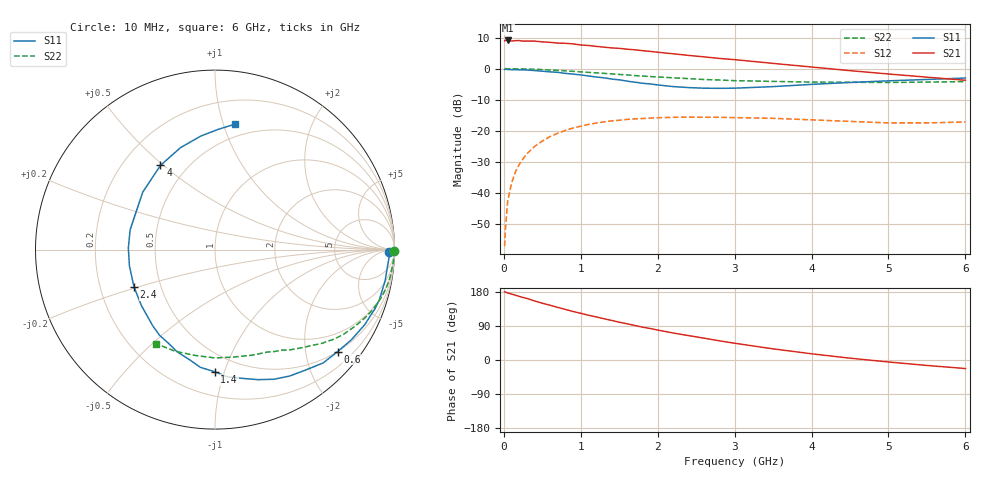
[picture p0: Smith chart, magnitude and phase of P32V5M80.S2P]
! SIEMENS Small Signal Semiconductors
! BFP181
! Si NPN RF Bipolar Junction Transistor in SOT143
! VCE = 2.5 V  IC = 0.8 mA
! Common Emitter S-Parameters:  March  1996
# GHz  S  MA  R  50
!  f  S11  S21  S12  S22
! GHz  MAG  ANG  MAG  ANG  MAG  ANG  MAG  ANG
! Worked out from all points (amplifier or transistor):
!   36 points, 10 MHz to 6 GHz, reference 50 ohm
!   highest |S21| = 9.1 dB at 50 MHz (marker M1)
!   |S21| within 3 dB of that: start of sweep to 1.697 GHz
!   unconditionally stable (mu >= 1): 3.36 GHz to end of sweep
!   at 250 MHz: K = 0.08, MSG = 18.9 dB, |S12| = -29.0 dB
!   at 1.4 GHz: K = 0.47, MSG = 11.7 dB, |S12| = -16.8 dB
!   at 6 GHz: K = 1.33, MAG = 3.3 dB, |S12| = -17.1 dB
!   S11 on the Smith chart (normalised r, x): 10 MHz: 54, -24; 600 MHz: 0.50, -2.68; 1.4 GHz: 0.37, -0.93; 2.4 GHz: 0.35, -0.19; 4 GHz: 0.36, +0.49; 6 GHz: 0.39, +1.09
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0.01  0.9696 -0.8  2.803 179.8  0.0014 87.9  0.999 -0.3
0.02  0.9785 -1.3  2.839 179.4  0.0026 91.6  0.9995 -0.7
0.05  0.97 -2.9  2.841 177.0  0.0074 90.7  0.9974 -1.6
0.1  0.9644 -6.8  2.782 174.1  0.0144 85.0  0.9969 -3.2
0.15  0.964 -10.2  2.816 171.0  0.0218 82.7  0.9943 -4.7
0.2  0.959 -13.4  2.827 167.9  0.0288 81.0  0.9914 -6.4
0.4  0.933 -26.7  2.776 155.8  0.0562 72.2  0.9776 -12.6
0.6  0.8887 -39.8  2.651 144.5  0.0809 63.2  0.9526 -18.4
0.8  0.84 -53.0  2.559 133.4  0.1018 54.8  0.9227 -23.8
0.9  0.8174 -59.6  2.499 128.1  0.1111 51.0  0.9044 -26.4
1.1  0.7631 -71.7  2.359 118.1  0.1268 43.9  0.8713 -31.2
1.4  0.6807 -90.1  2.156 104.5  0.1446 34.3  0.8243 -37.6
1.5  0.661 -97.1  2.123 99.8  0.1481 31.7  0.8064 -39.3
1.8  0.5828 -116.4  1.949 86.8  0.1579 24.2  0.7613 -44.4
2.2  0.515 -142.8  1.735 71.3  0.165 15.4  0.7127 -50.9
2.4  0.4967 -155.4  1.634 64.4  0.1664 11.4  0.6923 -54.0
3  0.4855 166.8  1.396 44.2  0.1633 2.3  0.6415 -62.8
3.5  0.5144 141.5  1.216 29.4  0.159 -2.8  0.6238 -70.5
4  0.5591 122.9  1.063 16.4  0.1503 -6.4  0.6081 -79.7
4.5  0.5996 108.7  0.929 4.8  0.1419 -8.5  0.6037 -89.9
5.5  0.6705 88.4  0.73 -14.4  0.1342 -4.5  0.6082 -111.2
6  0.707 81.1  0.651 -22.5  0.1389 -2.5  0.619 -122.3
